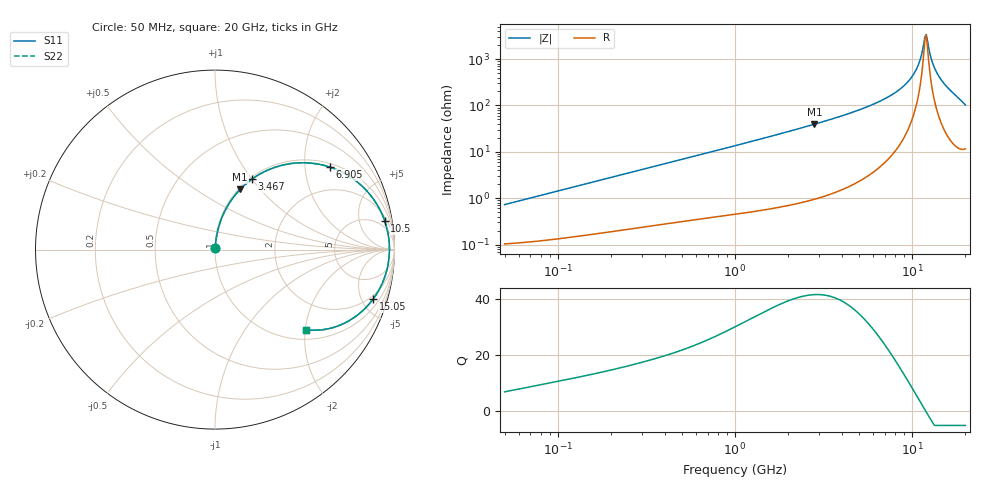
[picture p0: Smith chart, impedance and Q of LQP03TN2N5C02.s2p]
!Murata Part Number: LQP03TN2N5C02
!These Parameters are Measured in Series Mode Connection
!  o--[Z]--o
!Port1  Port2
!  o-------o
!Freq. Start=50[MHz] Stop=20[GHz], 401[Steps]
# Hz S RI R 50
!Freq.(Hz) S11(Real) S11(Imag) S21(Real) S21(Imag) S12(Real) S12(Imag) S22(Real) S22(Imag)
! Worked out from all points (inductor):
!   401 points, 50 MHz to 20 GHz, reference 50 ohm
!   read as one part in series: L = 2.28 nH near 51.52 MHz
!   highest Q = 41.6 at 2.811 GHz (marker M1), where L = 2.23 nH
!   self-resonance near 11.84 GHz
!   S11 on the Smith chart (normalised r, x): 50 MHz: 1.00, +0.01; 3.467 GHz: 1.02, +1.00; 6.905 GHz: 1.11, +2.70; 10.5 GHz: 3, +11; 15.05 GHz: 1.64, -6.10; 20 GHz: 1.23, -2.02
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5e7  0.00108 0.00718  0.9989 -0.00718  0.9989 -0.00718  0.00108 0.00718
1.364002e8  0.00191 0.0192  0.9981 -0.0192  0.9981 -0.0192  0.00191 0.0192
3.721004e8  0.00522 0.0506  0.9948 -0.0506  0.9948 -0.0506  0.00522 0.0506
1e9  0.0221 0.1314  0.9779 -0.1314  0.9779 -0.1314  0.0221 0.1314
2.728004e9  0.1328 0.3275  0.8672 -0.3275  0.8672 -0.3275  0.1328 0.3275
2.810964e9  0.1403 0.3355  0.8597 -0.3355  0.8597 -0.3355  0.1403 0.3355
3.466789e9  0.2058 0.3923  0.7942 -0.3923  0.7942 -0.3923  0.2058 0.3923
5.194772e9  0.4166 0.4784  0.5834 -0.4784  0.5834 -0.4784  0.4166 0.4784
6.905011e9  0.6399 0.4599  0.3601 -0.4599  0.3601 -0.4599  0.6399 0.4599
7.442007e9  0.7045 0.4334  0.2955 -0.4334  0.2955 -0.4334  0.7045 0.4334
9.178299e9  0.8722 0.2957  0.1278 -0.2957  0.1278 -0.2957  0.8722 0.2957
1.050288e10  0.9461 0.1582  0.0539 -0.1582  0.0539 -0.1582  0.9461 0.1582
1.115139e10  0.9644 0.0876  0.0356 -0.0876  0.0356 -0.0876  0.9644 0.0876
1.166392e10  0.9711 0.0322  0.0289 -0.0322  0.0289 -0.0322  0.9711 0.0322
1.201863e10  0.9719 -0.00536  0.0281 0.00536  0.0281 0.00536  0.9719 -0.00536
1.220001e10  0.9712 -0.0243  0.0288 0.0243  0.0288 0.0243  0.9712 -0.0243
1.276073e10  0.9645 -0.0811  0.0355 0.0811  0.0355 0.0811  0.9645 -0.0811
1.334722e10  0.9508 -0.1372  0.0492 0.1372  0.0492 0.1372  0.9508 -0.1372
1.417136e10  0.9217 -0.2093  0.0783 0.2093  0.0783 0.2093  0.9217 -0.2093
1.504638e10  0.8805 -0.2763  0.1195 0.2763  0.1195 0.2763  0.8805 -0.2763
1.774144e10  0.7054 -0.4172  0.2946 0.4172  0.2946 0.4172  0.7054 -0.4172
2e10  0.5083 -0.446  0.4917 0.446  0.4917 0.446  0.5083 -0.446
